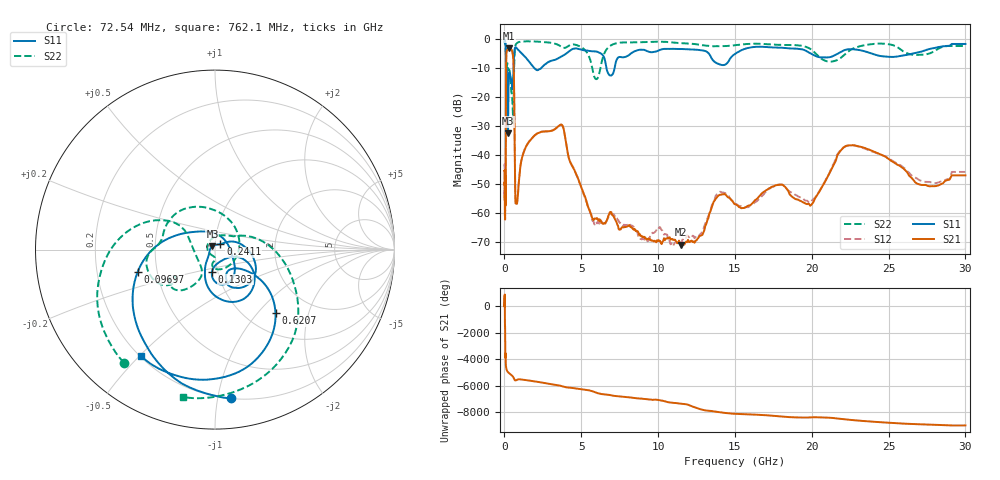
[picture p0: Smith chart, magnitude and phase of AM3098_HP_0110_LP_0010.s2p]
! Date/Time: Thu, Feb 28, 2019 8:37 AM
! Network Analyzer: Agilent Technologies E8364B Rev: A.07.50.67
! Sweep from 0.010 to 30.000 GHz, 1601 Points, Sweep Type: LOG
! Power Supply: 5.022 V, 0.002 A
# Hz S DB R 50
!freq MagS11 AngS11 MagS21 AngS21 MagS12 AngS12 MagS22 AngS22
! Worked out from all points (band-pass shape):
!   1601 points, 10 MHz to 30 GHz, reference 50 ohm
!   highest |S21| = -3.05 dB at 266.5 MHz (marker M1); lowest = -70.8 dB at 11.48 GHz (marker M2)
!   |S21| within 3 dB of the highest: 117.2 MHz to 563 MHz (445.8 MHz wide, 131 % of centre)
!   lowest |S11| = -32.4 dB at 231.6 MHz (marker M3), VSWR 1.05, Z = 48.6 + j1.87 ohm
!   |S11| at or under -10 dB: 175.1 MHz to 588.2 MHz (413.1 MHz wide, 108 % of centre); 1.967 GHz to 2.379 GHz (412 MHz wide, 19 % of centre); 6.642 GHz to 7.165 GHz (522.6 MHz wide, 7.57 % of centre)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
!   |S22| runs from -28.9 to -0.5 dB; largest |S21 - S12| = 0.011
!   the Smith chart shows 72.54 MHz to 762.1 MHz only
!   S11 on the Smith chart (normalised r, x): 72.54 MHz: 0.20, -1.09; 96.97 MHz: 0.39, -0.12; 130.3 MHz: 0.94, -0.23; 241.1 MHz: 1.06, +0.06; 620.7 MHz: 1.35, -1.25; 762.1 MHz: 0.20, -0.51
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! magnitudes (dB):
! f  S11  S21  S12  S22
! 10 MHz  -0.3  -45.5  -43.8  -0.5
! 38.04 MHz  -0.5  -58.9  -58.9  -0.8
! 72.54 MHz  -1.6  -53.9  -52.7  -1.8
! 96.97 MHz  -7.0  -24.5  -24.6  -8.0
! 130.3 MHz  -18.2  -4.7  -4.7  -10.5
! 144.7 MHz  -18.6  -3.9  -3.9  -11.2
! 185.8 MHz  -10.9  -3.6  -3.6  -8.2
! 231.6 MHz  -32.4  -3.2  -3.1  -9.9
! 241.1 MHz  -27.4  -3.1  -3.1  -10.1
! 266.5 MHz  -15.8  -3.1  -3.0  -10.4
! 550.5 MHz  -15.0  -5.4  -5.4  -25.1
! 620.7 MHz  -6.2  -14.3  -14.2  -12.2
! 699.9 MHz  -2.8  -52.6  -52.1  -2.5
! 762.1 MHz  -2.8  -56.2  -56.1  -1.5
! 2.084 GHz  -10.5  -32.5  -32.6  -0.7
! 3.723 GHz  -5.8  -29.4  -29.4  -2.6
! 5.812 GHz  -4.1  -62.3  -63.1  -12.3
! 7.926 GHz  -5.9  -64.6  -64.0  -1.0
! 11.48 GHz  -3.3  -70.8  -70.3  -1.3
! 19.8 GHz  -4.5  -56.6  -56.2  -3.0
! 22.67 GHz  -3.4  -36.5  -36.5  -3.2
! 30 GHz  -1.6  -46.9  -45.7  -2.3
